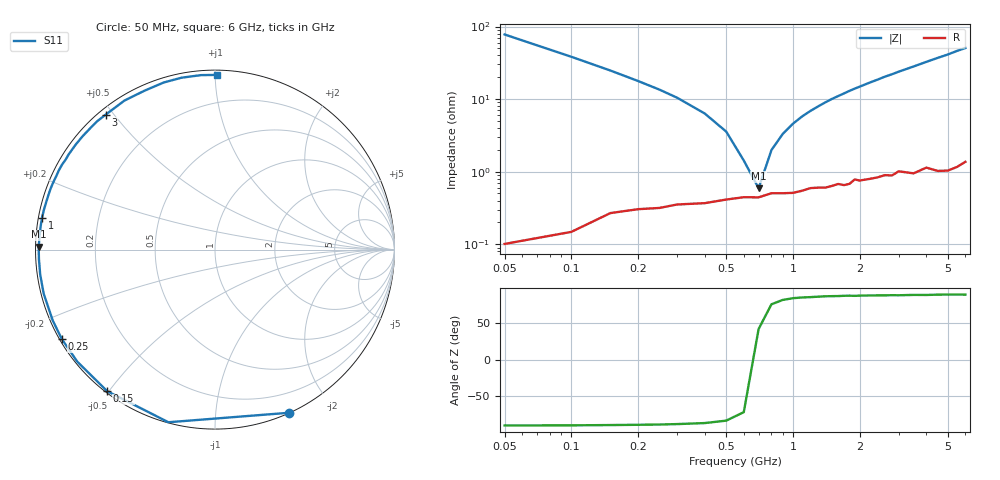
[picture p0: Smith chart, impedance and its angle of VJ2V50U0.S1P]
! Infineon Technologies  Discrete & RF Semiconductors
! BB 914
! Si Tuning Diode in SOT23
! VR = 2.5 V
! S-Parameters:  July  1999
# GHz  S  MA  R  50
!  f  S11
! GHz  MAG  ANG
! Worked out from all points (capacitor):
!   34 points, 50 MHz to 6 GHz, reference 50 ohm
!   read as one part to ground: C = 40.7 pF near 50 MHz
!   lowest |Z| = 592 mohm at 700 MHz (marker M1)
!   series resonance near 677.5 MHz, so ESL is about 1.4 nH
!   S11 on the Smith chart (normalised r, x): 50 MHz: 0.00, -1.55; 150 MHz: 0.01, -0.50; 250 MHz: 0.01, -0.27; 1 GHz: 0.01, +0.09; 3 GHz: 0.02, +0.48; 6 GHz: 0.03, +1.01
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0.05  0.9988 -65.5
0.1  0.9963 -105.1
0.15  0.9914 -127.3
0.2  0.9893 -140.9
0.25  0.9883 -149.8
0.3  0.9866 -156.4
0.4  0.9856 -165.6
0.5  0.9837 -171.9
0.6  0.9824 -176.9
0.7  0.9825 179.1
0.8  0.9801 175.6
1  0.98 169.6
1.1  0.9787 166.9
1.4  0.9769 159.6
1.6  0.9745 155.2
1.8  0.9749 150.9
2  0.9726 147.0
2.2  0.9719 143.1
2.4  0.9711 139.5
2.6  0.9698 135.7
2.8  0.9707 132.5
3  0.9676 129.0
3.5  0.9716 121.3
4  0.9686 113.8
4.5  0.9739 107.0
5  0.9757 101.0
5.5  0.9752 94.6
6  0.9733 89.4
